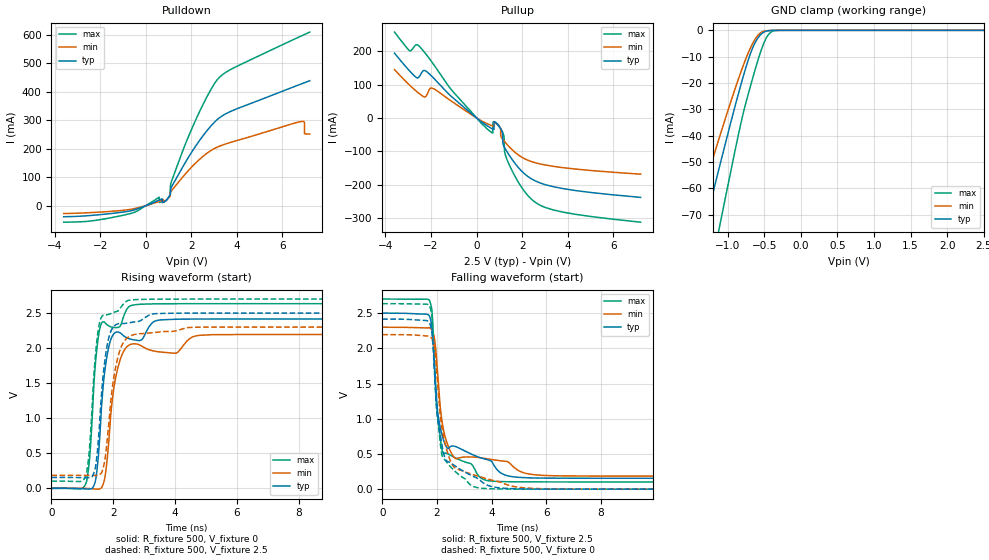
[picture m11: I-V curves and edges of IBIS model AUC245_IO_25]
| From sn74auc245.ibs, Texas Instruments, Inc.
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[Model]   AUC245_IO_25
Model_type  3-state
Enable   Active-Low
Vref =   0
Rref =   500
Cref =   30p
Vmeas =   1.25
| variable   typ   min   max
C_comp   6.41pF   5.69pF   6.76pF
| C_pullup   8.39pF   3.19pF   12.88pF
| C_pulldown   7.72pF   5.91pF   16.50pF
| C_tri-state   6.41pF   5.69pF   6.76pF
[Temperature Range]   40   100   -40
| Ambient temperature   25   85   -40
[Voltage range]   2.5   2.3   2.7
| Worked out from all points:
|   slope of the pulldown table from 0 to 0.375 V, typ, clamps not added: 30.7 ohm
|   slope of the pullup table from 0 to 0.375 V, typ, clamps not added: 19.3 ohm
|   GND clamp passes 1 mA (typ) near -0.52 V on its own axis
|   rising waveform, R_fixture 500, V_fixture 0: 20-80 % time 294ps typ, 364ps min, 249ps max; typ from 0 V to 2.42 V
|   falling waveform, R_fixture 500, V_fixture 2.5: 20-80 % time 445ps typ, 436ps min, 289ps max; typ from 2.5 V to 0.155 V
|   rising waveform, R_fixture 500, V_fixture 2.5: 20-80 % time 293ps typ, 369ps min, 249ps max; typ from 0.154 V to 2.5 V
|   falling waveform, R_fixture 500, V_fixture 0: 20-80 % time 390ps typ, 481ps min, 296ps max; typ from 2.42 V to 0 V
[GND Clamp]
| AUC245_IO_25
|   Voltage   I(typ)   I(min)   I(max)
-3.6V     -336.3mA   -280.4mA   -411.7mA
-1.51V    -96.49mA   -77.03mA   -129.3mA
-1.45V    -89.67mA   -71.42mA   -121.1mA
-1.29V    -71.61mA   -56.63mA   -99.1mA
-1.1V     -50.45mA   -39.48mA   -72.99mA
-850mV    -23.71mA   -18.22mA   -39.14mA
-725mV    -11.76mA   -8.97mA    -24.81mA
-620mV    -4.411mA   -3.121mA   -14.45mA
-520mV    -951.5uA   -506.2uA   -5.863mA
-435mV    -129.5uA   -70.83uA   -1.353mA
-320mV    -4.562uA   -5.052uA   -39.64uA
2.5V      1.104nA    235.6nA    1.576nA
[Pulldown]
| AUC245_IO_25
|   Voltage   I(typ)   I(min)   I(max)
-3.6V     -38.75mA   -27.46mA   -57.79mA
-1.145V   -23.84mA   -17.22mA   -36.09mA
590mV     19.92mA    14.98mA    30.03mA
600mV     20.28mA    15.25mA    11.17mA
910mV     19.98mA    20.14mA    19.19mA
1.14V     67.22mA    53.43mA    87.3mA
1.925V    176.6mA    128mA      252.2mA
3.16V     303.8mA    206.4mA    444.2mA
6.825V    427.5mA    295.7mA    595.8mA
6.965V    431.8mA    292.9mA    601mA
6.97V     431.9mA    252.6mA    601.2mA
7.2V      438.8mA    251.8mA    609.5mA
[Pullup]
| AUC245_IO_25
|   Voltage   I(typ)   I(min)   I(max)
-3.6V     193.7mA    144.6mA    256.9mA
-2.935V   140.5mA    97.95mA    200.9mA
-2.49V    125.8mA    71.54mA    212.7mA
-1.91V    120.8mA    88.21mA    162.4mA
445mV     -22.7mA    -16.54mA   -31.6mA
945mV     -21.56mA   -22.07mA   -19.39mA
1.14V     -42.13mA   -63.07mA   -43.86mA
1.19V     -82.98mA   -67.32mA   -51.19mA
1.235V    -89.26mA   -71.06mA   -103.2mA
1.455V    -113.7mA   -87.91mA   -143.1mA
2.52V     -186.4mA   -132.8mA   -249.6mA
7.2V      -237.6mA   -168.2mA   -311.9mA
[Ramp]
| AUC245_IO_25
| variable   typ   min   max
dV/dt_r   1.46/2.95E-10   1.32/3.66E-10   1.59/2.54E-10
dV/dt_f   1.41/4.55E-10   1.27/4.44E-10   1.56/2.99E-10
R_load = 500
[Rising Waveform]
| AUC245_IO_25
R_fixture =   500
C_fixture =   0
L_fixture =   0
V_fixture =   0
V_fixture_min = 0
V_fixture_max = 0
|   Time   V(typ)   V(min)   V(max)
0s        14.66nV    42.2nV     3.041nV
1.13ns    -8.448mV   -1.232mV   83.37mV
1.25ns    -9.66mV    -3.849mV   504.5mV
1.425ns   103.6mV    -9.837mV   1.78V
1.63ns    1.212V     13.64mV    2.36V
1.835ns   1.973V     554.8mV    2.323V
2.095ns   2.228V     1.614V     2.293V
2.665ns   2.119V     2.063V     2.617V
3.99ns    2.412V     1.927V     2.633V
34.99ns   2.416V     2.195V     2.634V
[Falling Waveform]
| AUC245_IO_25
R_fixture =   500
C_fixture =   0
L_fixture =   0
V_fixture =   2.5
V_fixture_min = 2.3
V_fixture_max = 2.7
|   Time   V(typ)   V(min)   V(max)
0s        2.5V       2.3V       2.7V
1.715ns   2.469V     2.292V     2.69V
1.815ns   2.32V      2.267V     2.552V
1.915ns   1.706V     2.133V     1.724V
2.03ns    1.09V      1.631V     1.032V
2.205ns   745.8mV    920.3mV    529.4mV
2.665ns   606.9mV    439.4mV    446.4mV
3.83ns    420.1mV    432.3mV    123.8mV
5.53ns    159.5mV    206mV      103.3mV
34.99ns   154.5mV    184.4mV    102.7mV
[Rising Waveform]
| AUC245_IO_25
R_fixture =   500
C_fixture =   0
L_fixture =   0
V_fixture =   2.5
V_fixture_min = 2.3
V_fixture_max = 2.7
|   Time   V(typ)   V(min)   V(max)
0s        154.5mV    184.4mV    102.6mV
1.13ns    150.7mV    184.2mV    201.8mV
1.24ns    152.8mV    183.4mV    612.6mV
1.425ns   297.4mV    182.9mV    1.898V
1.62ns    1.333V     218.4mV    2.442V
1.75ns    1.89V      467.3mV    2.472V
1.915ns   2.231V     1.22V      2.491V
2.175ns   2.349V     1.909V     2.538V
2.515ns   2.361V     2.165V     2.684V
34.99ns   2.5V       2.3V       2.7V
[Falling Waveform]
| AUC245_IO_25
R_fixture =   500
C_fixture =   0
L_fixture =   0
V_fixture =   0
V_fixture_min = 0
V_fixture_max = 0
|   Time   V(typ)   V(min)   V(max)
0s        2.416V     2.195V     2.634V
1.715ns   2.377V     2.174V     2.616V
1.815ns   2.233V     2.142V     2.47V
1.915ns   1.635V     1.994V     1.707V
1.99ns    1.17V      1.685V     1.133V
2.19ns    615.4mV    860.2mV    475.7mV
2.595ns   348mV      327.2mV    278.7mV
3.49ns    151.6mV    186.4mV    20.78mV
6.15ns    1.087mV    4.569mV    278uV
34.99ns   55.13uV    58.2uV     12.85uV
